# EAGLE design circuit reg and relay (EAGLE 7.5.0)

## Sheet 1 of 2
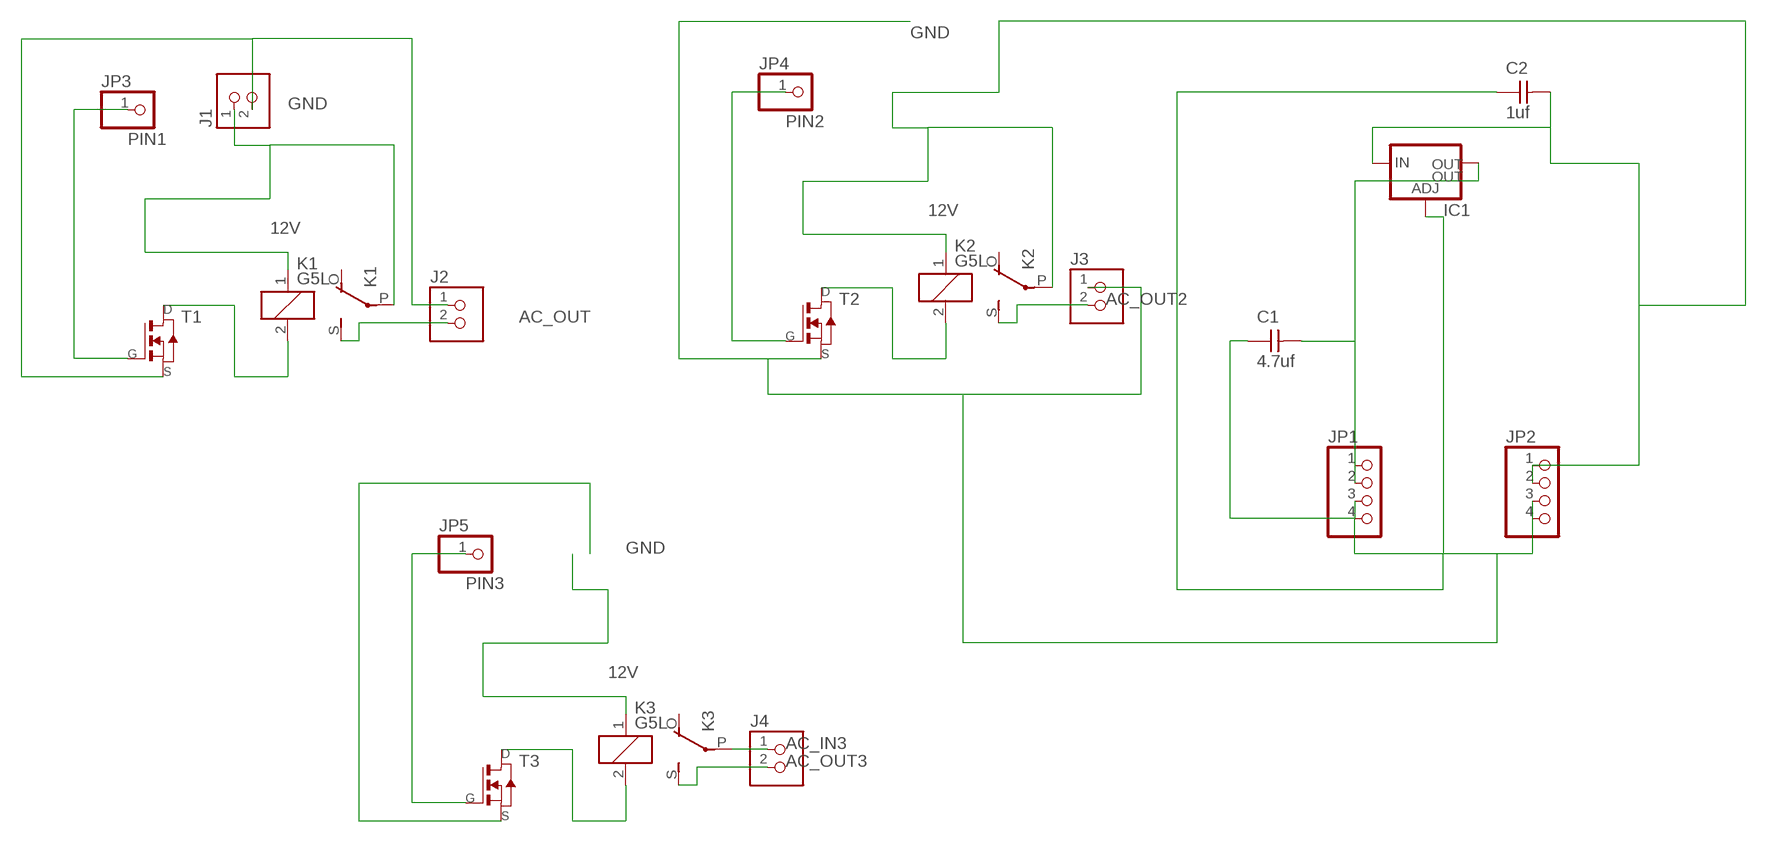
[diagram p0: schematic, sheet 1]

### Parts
C1  4.7uf  CAP-UNPOLARIZEDFAB  [C1206FAB]
C2  1uf  CAP-UNPOLARIZEDFAB  [C1206FAB]
IC1  V_REG_LM1117SOT223  [SOT223]
J1  TERM-1X02-FABLAB  [ED555DS-2DS]
J2  TERM-1X02-FABLAB  [ED555DS-2DS]
J3  TERM-1X02-FABLAB  [ED555DS-2DS]
J4  TERM-1X02-FABLAB  [ED555DS-2DS]
JP1  PINHD-1X4  [1X04]
JP2  PINHD-1X4  [1X04]
JP3  PINHD-1X1  [1X01]
JP4  PINHD-1X1  [1X01]
JP5  PINHD-1X1  [1X01]
K1  G5L  [G5LE]
K2  G5L  [G5LE]
K3  G5L  [G5LE]
T1  NMOSFETSOT23  [SOT-23]
T2  NMOSFETSOT23  [SOT-23]
T3  NMOSFETSOT23  [SOT-23]

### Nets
12V: C2.2 IC1.3(IN) J1.1 JP2.1 JP2.2 K1.1 K1.P(2:P) K2.1 K2.P(2:P) K3.1
AC_IN3: J4.1 K3.P(2:P)
AC_OUT: J2.2 K1.S(2:S)
AC_OUT2: J3.2 K2.S(2:S)
AC_OUT3: J4.2 K3.S(2:S)
GND: C1.1 C2.1 IC1.1(ADJ) J1.2 J2.1 J3.1 JP1.3 JP1.4 JP2.3 JP2.4 T1.2(S) T2.2(S) T3.2(S)
N$1: K2.2 T2.1(D)
N$2: K1.2 T1.1(D)
N$3: K3.2 T3.1(D)
PIN1: JP3.1 T1.3(G)
PIN2: JP4.1 T2.3(G)
PIN3: JP5.1 T3.3(G)
VC_OUT: C1.2 IC1.2(OUT) IC1.4(OUT) JP1.1 JP1.2
Unconnected: K1.O(2:O) K2.O(2:O) K3.O(2:O)

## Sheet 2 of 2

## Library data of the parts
C1 C2 = fab:CAP-UNPOLARIZED
IC1 = fab:V_REG_LM1117: Voltage Regulator LM1117 Standard adjustable voltage regulator but in SMD form. Spark Fun Electronics SKU : COM-00595; PROD_ID: VREG-08170
J1-J4 = fab:TERM-1X02: 3.5mm terminal block, 2 positions ED555-2DS as found in the fablab inventory.
JP1 JP2 = pinhead:PINHD-1X4: PIN HEADER
JP3-JP5 = pinhead:PINHD-1X1: PIN HEADER
K1-K3 = relay:G5L: RELAY 1 x switch, 10 A/120 V AC, 8 A/30 V ADC, Omron; OC_FARNELL: unknown; OC_NEWARK: unknown
T1-T3 = fab:NMOSFET: MOS FET

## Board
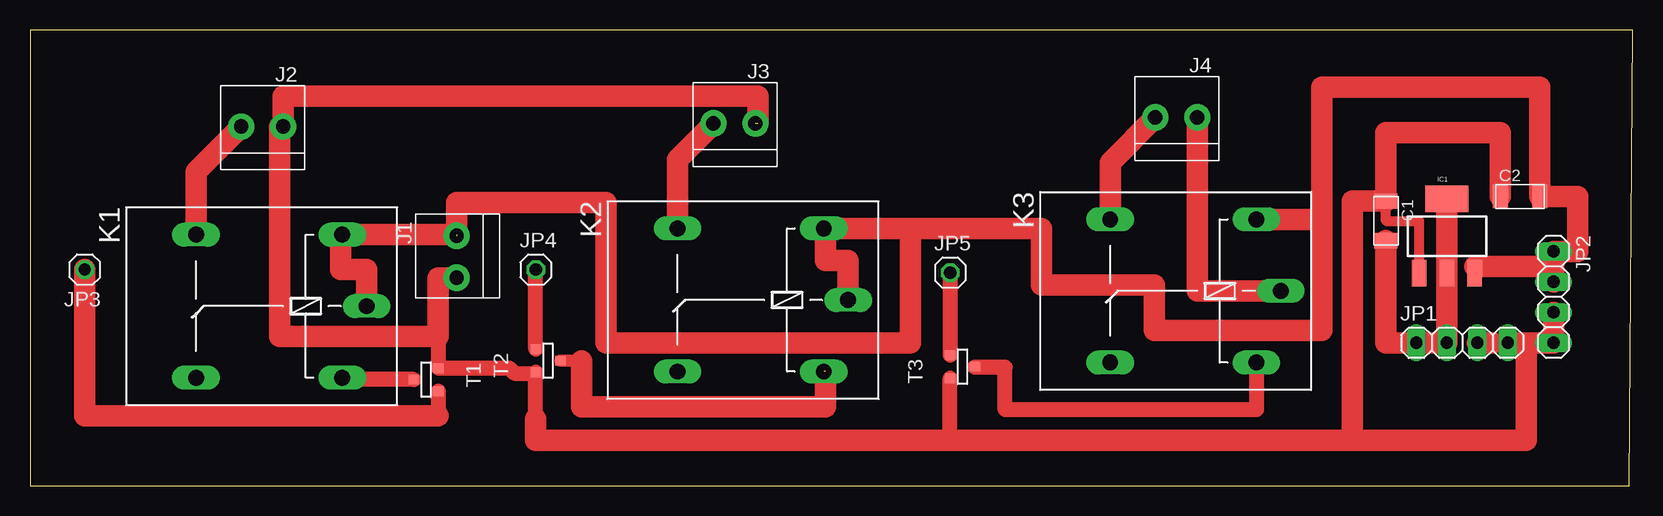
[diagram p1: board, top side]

Size 133.58 x 38.02 mm. Coordinates in mm from the lower left corner, seen from the top.
Outline: 0,0 133.33,0 133.58,38.02 0,38.02 0,0
Copper layers (1*16): Top 0.035mm / dielectric 1.5mm / Bottom 0.035mm
Design rules "default": minimum track width 10mil, minimum drill 24mil, track to track 8mil, track to pad 8mil, pad to pad 8mil, via to via 8mil, smd to smd 8mil, copper to edge 40mil, drill to drill 8mil, minimum pad ring 10mil, minimum via ring 8mil, stop-mask expansion 4mil, vias tented up to drill 0mil, thermal gap 10mil

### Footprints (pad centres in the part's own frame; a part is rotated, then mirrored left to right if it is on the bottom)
C1206FAB = smd 1.27 x 1.905: 1 -1.651,0; 2 1.651,0
SOT223 = smd 1.219 x 2.235: 1 -2.311,-3.099; 2 0,-3.099; 3 2.311,-3.099 | smd 3.6 x 2.2: 4 0,3.099
ED555DS-2DS = drill 1.2 pad 2.184: 1 1.8,0; 2 -1.7,0
1X04 = drill 1.016 long: 1 -3.81,0; 2 -1.27,0; 3 1.27,0; 4 3.81,0
1X01 = drill 1.016 octagon: 1 0,0
G5LE = drill 1.321 long: 1 -7.493,-5.969; 2 -7.493,5.969; O 4.699,5.969; P -9.525,0; S 4.699,-5.969
SOT-23 = smd 0.787 x 0.889: 1 0.025,-1.016; 2 -0.94,1.016; 3 0.991,1.016

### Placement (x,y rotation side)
C1  113.03,22.1 270 top
C2  124.21,24.13 0 top
IC1  118.11,20.83 0 top
J1  35.56,19.05 90 top
J2  19.3,29.97 0 top
J3  58.67,30.23 0 top
J4  95.5,30.73 0 top
JP1  119.38,11.94 0 top
JP2  127,15.75 270 top
JP3  4.57,18.03 180 top
JP4  42.16,18.03 0 top
JP5  76.71,17.78 0 top
K1  18.54,14.99 180 top
K2  58.67,15.49 180 top
K3  94.74,16.26 180 top
T1  33.02,8.89 270 top
T2  43.18,10.41 90 top
T3  77.72,9.91 90 top

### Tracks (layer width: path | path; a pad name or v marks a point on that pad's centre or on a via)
12V  (1 unrouted)
  Top 0.406: K1.1 25.91,20.96 | K2.1 66.29,21.46 | 127,18.29 JP2.1 | IC1.3 120.42,18.29 | C2.2 125.73,24.13 | 107.7,22.23 107.44,22.23
  Top 1.778: K1.1 35.56,20.96 | J1.1 35.56,23.62 48.01,23.62 48.01,11.94 73.41,11.94 73.41,21.46 | K3.1 107.44,22.23 | K2.1 73.41,21.46 | 73.41,21.46 84.33,21.46 84.33,16.76 93.73,16.76 93.73,12.95 107.7,12.95 107.7,22.23 107.7,33.27 125.86,33.27 C2.2 129.03,24.13 129.03,19.56 JP2.1 | 25.91,20.96 25.91,18.03 28.07,18.03 K1.P | 66.29,21.46 66.29,18.8 68.2,18.8 K2.P | JP2.2 127,18.29 120.42,18.29
AC_IN3
  Top 1.778: J4.1 97.3,16.26 K3.P
AC_OUT
  Top 1.778: J2.2 13.84,26.21 K1.S
AC_OUT2
  Top 1.778: J3.2 53.98,27.23 K2.S
AC_OUT3
  Top 1.778: J4.2 90.04,26.97 K3.S
GND  (1 unrouted)
  Top 0.406: JP1.4 121.92,11.94 | T3.2 76.71,4.32 | J2.1 20.83,29.97
  Top 0.813: IC1.1 115.8,22.1 113.03,22.1 C1.1
  Top 1.27: 42.16,5.59 T2.2 42.09,9.4 40.39,9.4 39.95,9.83 T1.2 34.04,12.45 | 76.71,3.81 T3.2
  Top 1.778: JP2.3 JP2.4 124.71,11.94 | JP1.3 121.92,11.94 | 110.24,3.81 110.24,23.75 C1.1 113.03,29.46 122.56,29.46 C2.1 | J1.2 34.04,17.35 34.04,12.45 20.83,12.45 20.83,29.97 | 60.71,30.23 60.71,32.51 21.1,32.51 J2.1 | 124.71,11.94 JP1.4 | 42.16,5.59 42.16,3.81 76.71,3.81 110.24,3.81 | 110.24,3.81 124.71,3.81 124.71,11.94
N$1  (1 unrouted)
  Top 1.016: 45.97,10.44 T2.1
  Top 1.778: 66.29,9.53 66.29,6.6 45.97,6.6 45.97,10.44
N$2
  Top 0.406: 26.19,8.87 K1.2
  Top 1.27: T1.1 26.19,8.87
N$3
  Top 0.406: T3.1 78.74,9.91
  Top 1.27: 78.74,9.91 81.28,9.91 81.28,6.35 102.24,6.35 K3.2
PIN1
  Top 1.27: T1.3 34.04,5.84
  Top 1.778: 34.04,5.84 4.57,5.84 JP3.1
PIN2
  Top 1.27: T2.3 JP4.1
PIN3
  Top 1.27: JP5.1 T3.3
VC_OUT
  Top 1.778: IC1.4 IC1.2 JP1.2 JP1.1 113.03,11.94 C1.2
